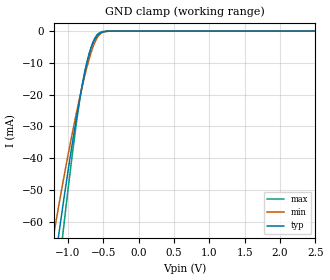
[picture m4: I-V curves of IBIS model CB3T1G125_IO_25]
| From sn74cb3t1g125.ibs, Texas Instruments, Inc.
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[Model]   CB3T1G125_IO_25
Model_type  Terminator
| variable   typ   min   max
C_comp   3.99pF   3.08pF   5.16pF
| C_tri-state   3.99pF   3.08pF   5.16pF
[Temperature Range]   40   100   -40
| Ambient temperature   25   85   -40
[Voltage range]   2.5   2.3   2.7
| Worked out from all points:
|   GND clamp passes 1 mA (typ) near -0.57 V on its own axis
[GND Clamp]
| CB3T1G125_IO_25
|   Voltage   I(typ)   I(min)   I(max)
-5.5V     -966.8mA   -814.4mA   -1.126A
-1.225V   -79.45mA   -67.08mA   -94.83mA
-1.18V    -72.07mA   -61.23mA   -85.5mA
-1.135V   -64.84mA   -55.51mA   -76.33mA
-1.11V    -60.89mA   -52.38mA   -71.31mA
-1.07V    -54.68mA   -47.46mA   -63.4mA
-895mV    -29.36mA   -27.32mA   -31.28mA
-790mV    -16.21mA   -16.63mA   -15.87mA
-680mV    -5.738mA   -7.302mA   -5.601mA
-570mV    -1.086mA   -1.527mA   -785.7uA
-415mV    -29.05uA   -40.98uA   -6.583uA
2.5V      184.6pA    1.99nA     62.62pA
